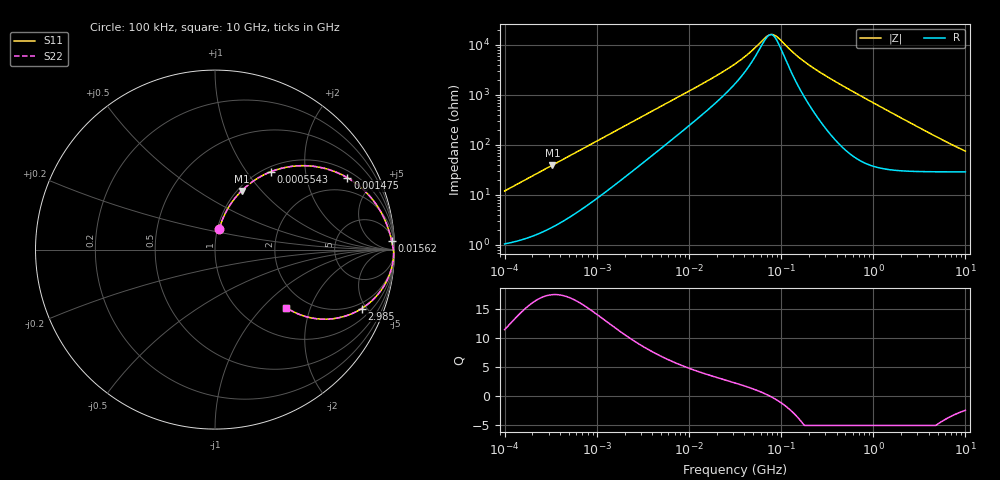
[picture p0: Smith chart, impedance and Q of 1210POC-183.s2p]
# MHz S MA R 50
!Freq  MagS11  AngS11  MagS21  AngS21  MagS12  AngS12  MagS22  AngS22
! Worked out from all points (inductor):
!   801 points, 100 kHz to 10 GHz, reference 50 ohm
!   read as one part in series: L = 19 uH near 105.9 kHz
!   highest Q = 17.4 at 330.2 kHz (marker M1), where L = 18.9 uH
!   self-resonance near 76.25 MHz
!   S11 on the Smith chart (normalised r, x): 100 kHz: 1.02, +0.24; 554.3 kHz: 1.08, +1.32; 1.475 MHz: 1.29, +3.49; 15.62 MHz: 11, +36; 2.985 GHz: 1.59, -4.64; 10 GHz: 1.58, -1.38
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0.1  0.1175 78.3  0.9829 -6.7  0.9829 -6.7  0.1175 78.3
0.1966754  0.2253 73.4  0.9603 -13.0  0.9603 -13.0  0.2253 73.4
0.3301794  0.3592 65.7  0.9129 -21.0  0.9129 -21.0  0.3592 65.7
0.5543065  0.5363 54.2  0.8125 -32.4  0.8125 -32.4  0.5363 54.2
0.6878599  0.6148 48.5  0.7509 -37.8  0.7509 -37.8  0.6148 48.5
0.9857119  0.7356 38.7  0.6274 -47.2  0.6274 -47.2  0.7356 38.7
1.474857  0.8393 28.5  0.4789 -56.8  0.4789 -56.8  0.8393 28.5
2.475996  0.9181 18.1  0.3125 -65.9  0.3125 -65.9  0.9181 18.1
4.663908  0.9608 9.9  0.174 -72.1  0.174 -72.1  0.9608 9.9
15.62248  0.9852 2.9  0.0525 -72.2  0.0525 -72.2  0.9852 2.9
31.62278  0.9902 1.2  0.02377 -65.1  0.02377 -65.1  0.9902 1.2
45.31584  0.992 0.7  0.01432 -55.5  0.01432 -55.5  0.992 0.7
68.78599  0.9935 0.1  0.006883 -19.0  0.006883 -19.0  0.9935 0.1
79.43282  0.9939 -0.1  0.00613 8.4  0.00613 8.4  0.9939 -0.1
91.72759  0.9943 -0.2  0.006974 35.5  0.006974 35.5  0.9943 -0.2
143.3013  0.9953 -0.8  0.01548 71.8  0.01548 71.8  0.9953 -0.8
217.5204  0.9957 -1.6  0.02773 80.3  0.02773 80.3  0.9957 -1.6
630.9573  0.9915 -5.1  0.08914 82.0  0.08914 82.0  0.9915 -5.1
1474.857  0.965 -11.8  0.2048 74.3  0.2048 74.3  0.965 -11.8
2985.383  0.8802 -21.9  0.3767 60.8  0.3767 60.8  0.8802 -21.9
5385.797  0.7235 -32.4  0.5495 44.9  0.5495 44.9  0.7235 -32.4
10000  0.5125 -39.1  0.6839 28.2  0.6839 28.2  0.5125 -39.1
